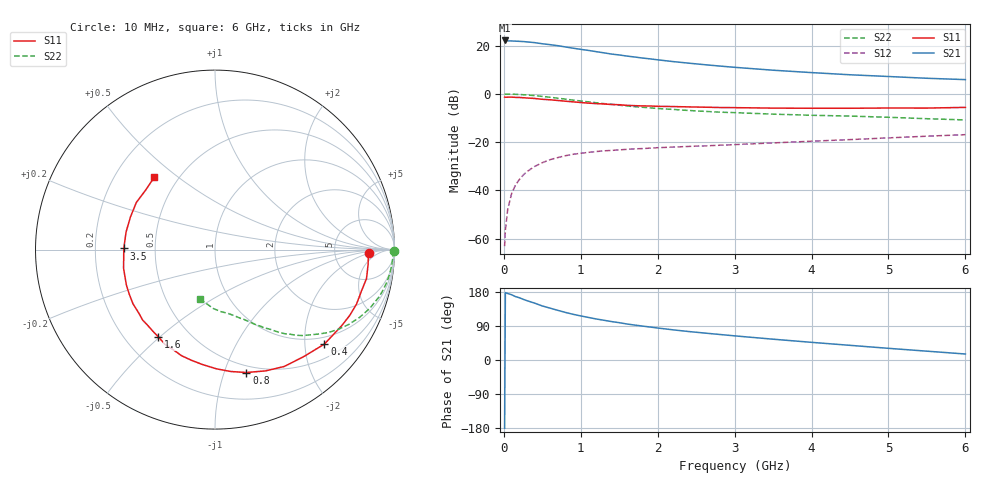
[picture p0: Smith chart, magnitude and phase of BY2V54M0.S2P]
! SIEMENS Small Signal Semiconductors
! BFY420
! Si NPN RF SIEGET Grounded Emitter Transistor in MICRO-X
! VCE = 2.5 V  IC = 4 mA
! Common Emitter S-Parameters:  October  1996
# GHz  S  MA  R  50
!  f  S11  S21  S12  S22
! GHz  MAG  ANG  MAG  ANG  MAG  ANG  MAG  ANG
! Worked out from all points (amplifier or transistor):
!   36 points, 10 MHz to 6 GHz, reference 50 ohm
!   highest |S21| = 22.2 dB at 10 MHz (marker M1)
!   |S21| within 3 dB of that: start of sweep to 860.2 MHz
!   unconditionally stable (mu >= 1): 3.366 GHz to end of sweep
!   at 250 MHz: K = 0.10, MSG = 27.7 dB, |S12| = -33.7 dB
!   at 1.4 GHz: K = 0.46, MSG = 20.0 dB, |S12| = -23.4 dB
!   at 6 GHz: K = 1.16, MAG = 9.0 dB, |S12| = -16.9 dB
!   S11 on the Smith chart (normalised r, x): 10 MHz: 13, -2; 400 MHz: 0.82, -2.45; 800 MHz: 0.44, -1.19; 1.6 GHz: 0.34, -0.49; 3.5 GHz: 0.33, +0.01; 6 GHz: 0.37, +0.41
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0.01  0.8594 -1.2  12.83 -180.0  0.0007 83.2  0.9953 -0.5
0.02  0.8544 -2.3  12.76 177.9  0.0015 85.8  0.9903 -1.0
0.05  0.857 -5.4  12.56 175.4  0.004 85.8  0.9919 -2.7
0.1  0.8594 -10.8  12.53 172.3  0.0085 85.4  0.9874 -5.5
0.15  0.8481 -15.7  12.41 167.4  0.0128 80.1  0.9821 -8.2
0.25  0.8353 -26.1  12.18 160.3  0.0207 75.1  0.9634 -13.4
0.4  0.8054 -40.8  11.57 150.1  0.0314 68.7  0.9224 -20.8
0.5  0.7744 -50.4  10.96 142.6  0.0376 63.7  0.8891 -25.2
0.6  0.7567 -59.4  10.5 136.9  0.0434 59.8  0.8532 -29.3
0.7  0.732 -67.4  10.01 131.1  0.0479 56.4  0.8172 -33.0
0.8  0.7067 -75.7  9.411 125.6  0.0524 52.1  0.7807 -36.3
0.9  0.6846 -82.7  8.87 120.6  0.0561 49.4  0.7455 -39.1
1.1  0.6442 -96.2  7.978 112.3  0.0615 44.9  0.6843 -44.4
1.4  0.6041 -112.8  6.703 101.4  0.0675 40.0  0.6092 -50.3
1.6  0.5796 -123.0  6.087 95.0  0.0711 37.6  0.5637 -53.6
1.9  0.5629 -135.8  5.331 87.0  0.0753 35.3  0.5145 -57.9
2.2  0.5476 -146.6  4.681 79.6  0.0791 33.3  0.4773 -61.4
2.8  0.5232 -163.8  3.79 67.5  0.0864 31.4  0.4195 -67.7
3.5  0.5082 179.3  3.1 54.9  0.0966 29.8  0.3813 -74.2
4.5  0.5049 158.9  2.495 38.7  0.1131 26.9  0.3475 -84.5
5.5  0.5092 139.3  2.111 23.3  0.1331 22.5  0.3066 -98.3
6  0.5261 130.1  1.98 15.8  0.1432 19.9  0.2891 -106.8
